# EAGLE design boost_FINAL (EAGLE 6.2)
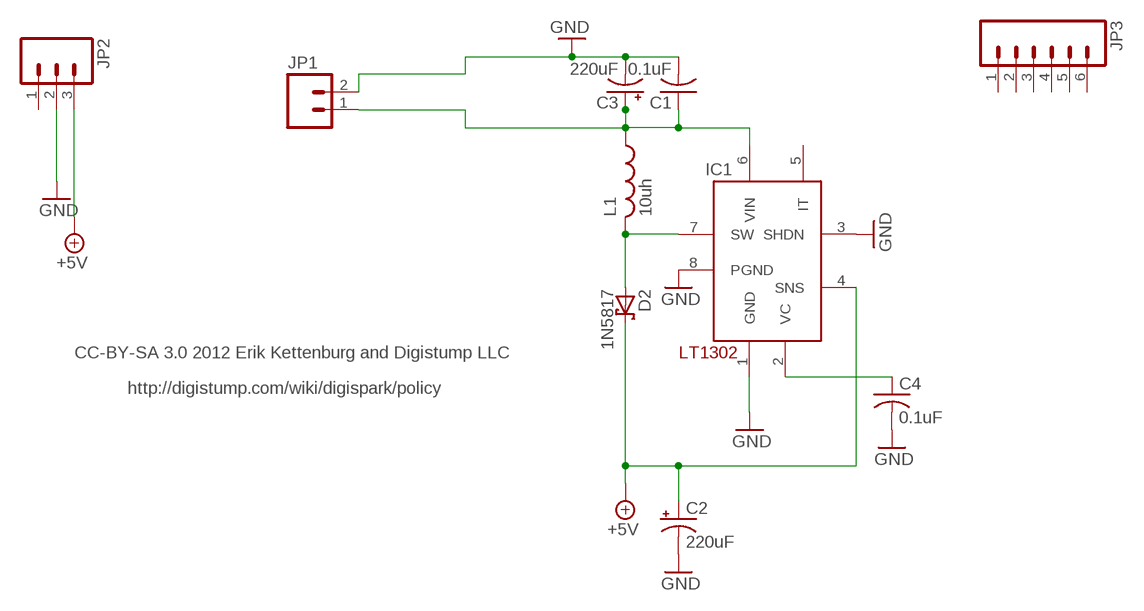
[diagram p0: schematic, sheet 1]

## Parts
C1  0.1uF  C-US025-024X044  [C025-024X044]
C2  220uF  CPOL-USE2.5-6  [E2,5-6]
C3  220uF  CPOL-USE2.5-6  [E2,5-6]
C4  0.1uF  C-US025-024X044  [C025-024X044]
D2  1N5817  SCHOTTKY-DIODEDO41  [DO41-10]
IC1  LT1302  [DIL08]
JP1  M023.5MM  [SCREWTERMINAL-3.5MM-2]
JP2  M03PTH  [1X03]
JP3  M06SIP  [1X06]
L1  10uh  L  [6000]

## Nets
+5V: C2.+ D2.C IC1.4(SNS) JP2.3
BATT+: C1.1 C3.+ IC1.6(VIN) JP1.1 L1.1
GND: C1.2 C2.- C3.- C4.2 IC1.1(GND) IC1.3(SHDN) IC1.8(PGND) JP1.2 JP2.2
N$4: C4.1 IC1.2(VC)
N$5: D2.A IC1.7(SW) L1.2
Unconnected: IC1.5(IT) JP2.1 JP3.1 JP3.2 JP3.3 JP3.4 JP3.5 JP3.6

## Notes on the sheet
- CC-BY-SA 3.0 2012 Erik Kettenburg and Digistump LLC
- http://digistump.com/wiki/digispark/policy

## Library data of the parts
C1 C4 = rcl-ez:C-US: CAPACITOR, American symbol
C2 C3 = rcl-ez:CPOL-US: POLARIZED CAPACITOR, American symbol
D2 = usbbuck:SCHOTTKY-DIODE: Schottky Diode
IC1 = usbbuck:LT1302
JP1 = SparkFun:M02: Header 2
JP2 = SparkFun:M03: Header 3 Standard 3-pin 0.1" header. Use with straight break away headers (SKU : PRT-00116), right angle break away headers (PRT-00553), swiss pins (PRT-00743), machine pins (PRT-00117), and female headers (PRT-00115). Molex polarized connector foot print use with SKU : PRT-08232 with associated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
JP3 = SparkFun:M06: Header 6 Standard 6-pin 0.1" header. Use with straight break away headers (SKU : PRT-00116), right angle break away headers (PRT-00553), swiss pins (PRT-00743), machine pins (PRT-00117), and female headers (PRT-00115). Molex polarized connector foot print use with SKU : PRT-08094 with associated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
L1 = usbbuck:L

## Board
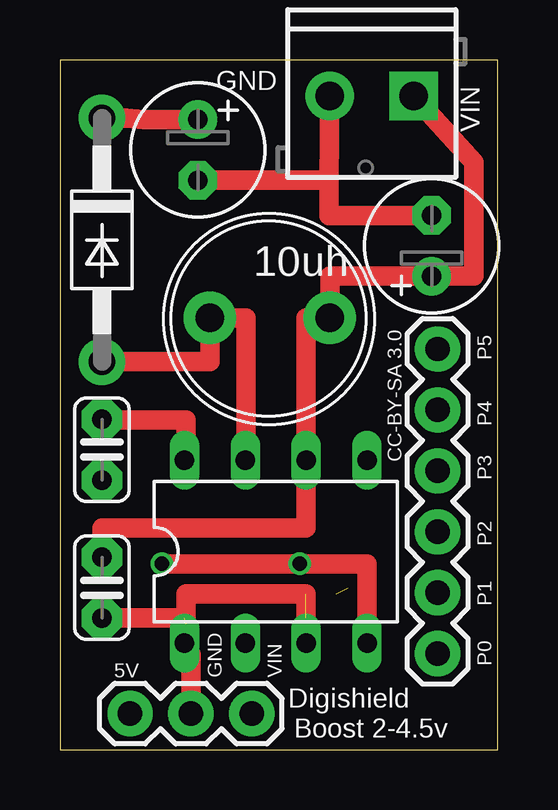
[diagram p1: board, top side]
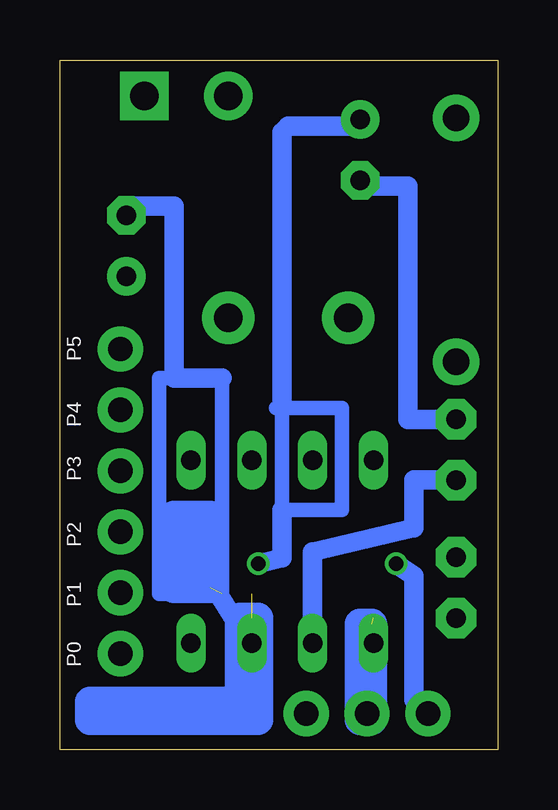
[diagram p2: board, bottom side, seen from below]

Size 18.25 x 28.75 mm. Coordinates in mm from the lower left corner, seen from the top.
Outline: 0,28.75 0,0 18.25,0 18.25,28.75 0,28.75
Copper layers (1*16): Top 0.0356mm / dielectric 1.5011mm / Bottom 0.0356mm
Design rules: minimum track width 8mil, minimum drill 13mil, track to track 12mil, track to pad 12mil, pad to pad 12mil, via to via 12mil, smd to smd 8mil, copper to edge 15mil, drill to drill 12mil, minimum pad ring 7mil, minimum via ring 7mil, stop-mask expansion 4mil, vias tented up to drill 50mil, thermal gap 10mil

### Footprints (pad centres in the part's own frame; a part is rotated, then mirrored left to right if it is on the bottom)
C025-024X044 = drill 0.813 pad 1.676 octagon: 1 -1.27,0; 2 1.27,0
E2,5-6 = drill 0.813 pad 1.6: + -1.27,0 | drill 0.813 pad 1.6 octagon: - 1.27,0
DO41-10 = drill 1.118 pad 1.93: A 5.08,0; C -5.08,0
DIL08 = drill 0.813 long: 1 -3.81,-3.81; 2 -1.27,-3.81; 3 1.27,-3.81; 4 3.81,-3.81; 5 3.81,3.81; 6 1.27,3.81; 7 -1.27,3.81; 8 -3.81,3.81
SCREWTERMINAL-3.5MM-2 = drill 1.2 pad 2.032 square: 1 0,0 | drill 1.2 pad 2.032: 2 3.5,0
1X03 = drill 1.016 pad 1.88: 1 0,0; 2 2.54,0; 3 5.08,0
1X06 = drill 1.016 pad 1.88: 1 0,0; 2 2.54,0; 3 5.08,0; 4 7.62,0; 5 10.16,0; 6 12.7,0
6000 = drill 1.2 pad 2.184: 1 -2.5,0; 2 2.5,0

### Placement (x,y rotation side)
C1  1.75,6.75 270 top
C2  5.75,25 270 top
C3  15.5,21 90 top
C4  1.75,12.5 90 top
D2  1.75,21.25 270 top
IC1  9,8.25 0 top
JP1  14.75,27.25 180 top
JP2  8,1.5 180 top
JP3  15.75,4 90 top
L1  8.75,18 180 top

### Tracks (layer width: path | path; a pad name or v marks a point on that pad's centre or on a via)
+5V  (via drill 0.6)
  Top 0.813: C2.+ 3.5,26.27 2.75,26.33 D2.C | v4.25,7.75 v10,7.75 12.81,7.75 IC1.4
  Bottom 0.203: C2.+ 5.79,25.96 5.79,26
  Bottom 0.61: 9,14.25 6.5,14.25 6.5,10 9,10 9,14.25 | 9.25,14.25 9,14.25
  Bottom 0.813: v4.25,7.75 3.5,7.25 3.5,2.08 JP2.3 | 5.75,26 5.79,26 8.75,26 9,25.75 9,14.25 | v10,7.75 9,8 9,10
BATT+
  Top 0.813: JP1.1 17.25,24.5 17.25,19.73 C3.+ 11.25,19.73 L1.1 10.27,18 IC1.6 10.27,9.25 9,9.25 1.75,9.23 C1.1
GND  (3 unrouted)
  Top 0.813: C2.- 11.21,23.73 | 11.21,23.73 JP1.2 | C1.2 5.19,5.48 IC1.1 5.25,4.44 | JP2.2 5.46,3.94 5.25,4.44 | 5.25,4.44 5.25,6.5 10.27,6.5 IC1.3 | C3.- 11.21,22.27 11.21,23.73 | IC1.8 5.25,12.06 5.25,13.75 1.75,13.75 C4.2
  Bottom 0.61: 11.5,6.5 11.5,15.5 14.13,15.5 14.13,6.5 11.5,6.5 | 11.5,6.5 11.5,6.25
  Bottom 0.813: C4.2 3.75,13.77 3.75,23.5 5.75,23.5 C2.- | 11.5,15.5 13.5,15.5 13.5,22.66 15.5,22.66 C3.- | 11.5,6.25 10.27,4.25 IC1.3
  Bottom 1.27: 12,6.75 13.5,6.75 13.5,9.75 12,9.75 12,7.5 12.75,7.5 12.75,8.75 | 10,5.5 10,1.25 17,1.25 17,2 10.25,2 10.25,5.5 10.75,5.5 10.75,2.5 | 5.25,5.25 5.25,1.25 5.75,1.25 5.75,5.25 5.25,5.25
N$4
  Bottom 0.813: C4.1 3.5,11.23 3.5,9.25 7.73,8.25 IC1.2
N$5
  Top 0.813: D2.A 6.25,16.17 L1.2 7.75,18 7.75,12.08 IC1.7

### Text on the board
tPlace: GND | VIN | CC-BY-SA 3.0 | 5V | GND | VIN | Digishield | Boost 2-4.5v
tNames: P5 | P4 | P3 | P2 | P1 | P0
bNames: P5 | P4 | P3 | P2 | P1 | P0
